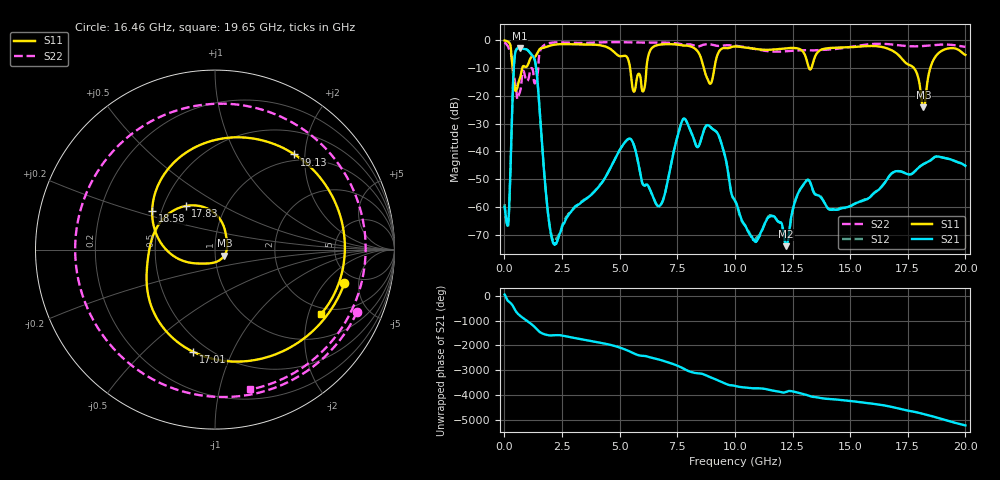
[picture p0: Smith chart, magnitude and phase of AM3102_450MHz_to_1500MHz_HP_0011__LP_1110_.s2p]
!Agilent Technologies,E8364B,MY43040894,A.07.50.67
!Agilent E8364B: A.07.50.67
!Date: Thursday, January 11, 2018 05:33:58
!Correction: S11(Full 2 Port(1,2))
!S21(Full 2 Port(1,2))
!S12(Full 2 Port(1,2))
!S22(Full 2 Port(1,2))
!S2P File: Measurements: S11, S21, S12, S22:
# Hz S  dB  R 50
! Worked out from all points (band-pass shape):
!   1601 points, 10 MHz to 20 GHz, reference 50 ohm
!   highest |S21| = -2.76 dB at 659.7 MHz (marker M1); lowest = -74.1 dB at 12.23 GHz (marker M2)
!   |S21| within 3 dB of the highest: 448.5 MHz to 1.245 GHz (796.9 MHz wide, 94.1 % of centre)
!   lowest |S11| = -24.2 dB at 18.18 GHz (marker M3), VSWR 1.13, Z = 55.4 - j3.66 ohm
!   |S11| at or under -10 dB: 5.453 GHz to 6.164 GHz (710.3 MHz wide, 12.2 % of centre); 8.648 GHz to 9.11 GHz (462.6 MHz wide, 5.21 % of centre); 17.77 GHz to 18.48 GHz (705.1 MHz wide, 3.89 % of centre)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
!   |S22| runs from -21.1 to -0.7 dB; largest |S21 - S12| = 0.0021
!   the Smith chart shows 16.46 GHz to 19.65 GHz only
!   S11 on the Smith chart (normalised r, x): 16.46 GHz: 3.96, -3.32; 17.01 GHz: 0.42, -0.72; 17.83 GHz: 0.65, +0.34; 18.58 GHz: 0.44, +0.23; 19.13 GHz: 0.88, +1.79; 19.65 GHz: 1.78, -2.43
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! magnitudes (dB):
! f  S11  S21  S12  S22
! 10 MHz  0.0  -60.0  -59.0  -0.7
! 172.4 MHz  -0.6  -65.2  -66.0  -2.5
! 434.8 MHz  -16.2  -6.9  -6.9  -13.8
! 659.7 MHz  -14.1  -2.8  -2.8  -19.0
! 1.347 GHz  -5.7  -8.2  -8.2  -15.3
! 2.109 GHz  -1.7  -72.9  -72.0  -0.8
! 3.346 GHz  -1.5  -58.2  -58.0  -1.0
! 5.42 GHz  -8.4  -35.4  -35.4  -0.8
! 6.682 GHz  -1.6  -59.8  -59.7  -0.8
! 7.794 GHz  -1.9  -28.2  -28.2  -1.6
! 10.01 GHz  -2.2  -57.7  -57.8  -1.9
! 12.23 GHz  -2.9  -74.1  -73.7  -3.9
! 13.34 GHz  -9.5  -52.9  -53.0  -3.6
! 16.46 GHz  -2.6  -51.7  -51.7  -1.3
! 16.68 GHz  -3.1  -49.1  -49.1  -1.4
! 17.01 GHz  -4.7  -47.1  -47.2  -1.7
! 17.83 GHz  -10.7  -47.0  -47.0  -2.2
! 18.18 GHz  -24.2  -44.6  -44.5  -2.0
! 18.58 GHz  -7.7  -42.6  -42.6  -1.8
! 19.13 GHz  -3.2  -42.4  -42.4  -1.5
! 19.65 GHz  -3.2  -43.8  -43.8  -1.9
! 20 GHz  -5.2  -45.2  -45.1  -2.3
